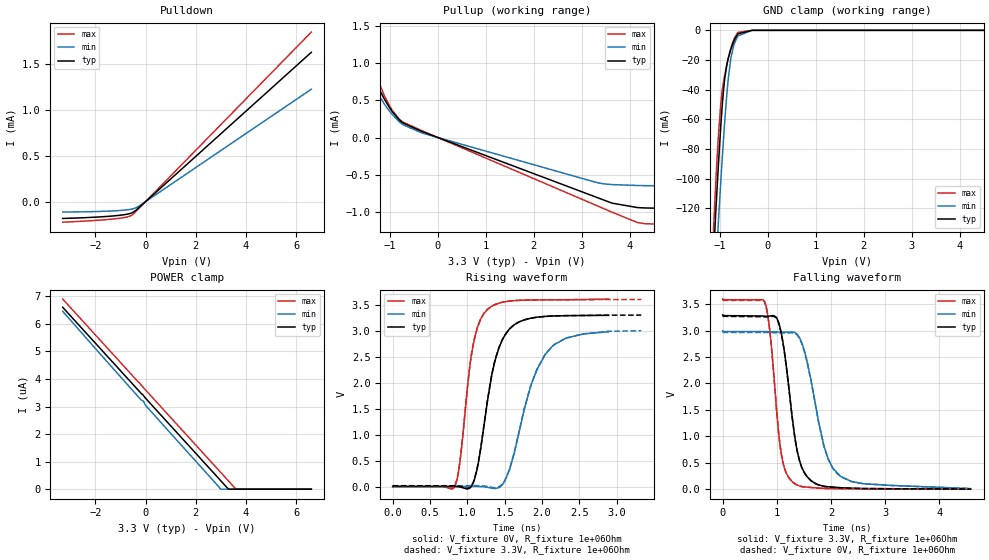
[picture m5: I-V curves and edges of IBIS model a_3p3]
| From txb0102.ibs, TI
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|   a_3p3 Model
[Model]   a_3p3
Model_type   I/O
Polarity   Non-Inverting
Enable   Active-High
Vinl = 1.155
Vinh = 2.145
Vmeas = 1.65
Vref = 0
Cref = 2pF
Rref = 1e6
|   typ   min   max
|   (nom PVT)   (fast PVT)   (slow PVT)
C_comp   3.766e-12   3.694e-12   3.795e-12
[Model spec]
|subparameter
Vinl   1.155   1.05   1.26
Vinh   2.145   1.95   2.34
| Where nom  PVT is Nominal Process, 3.3V, 27C
|   Fast PVT is Strong Process,  3.6V, -40C
|   Slow PVT is Weak Process,   3V, 125C
[Voltage Range]   3.3   3   3.6
|Junction Temperature
[Temperature Range]   27   125   -40
[Pullup Reference]   3.3   3   3.6
[Pulldown Reference]   0   0   0
[Power Clamp Reference]   3.3   3   3.6
[GND Clamp Reference]   0   0   0
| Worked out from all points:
|   slope of the pulldown table from 0 to 0.495 V, typ, clamps not added: 4.05 kohm
|   slope of the pullup table from 0 to 0.495 V, typ, clamps not added: 4.1 kohm
|   falling waveform, V_fixture 3.3V, R_fixture 1e+06Ohm: 20-80 % time 256ps typ, 373ps min, 193ps max; typ from 3.3 V to -0.003 V
|   rising waveform, V_fixture 0V, R_fixture 1e+06Ohm: 20-80 % time 245ps typ, 363ps min, 183ps max; typ from 0 V to 3.3 V
|   rising waveform, V_fixture 3.3V, R_fixture 1e+06Ohm: 20-80 % time 246ps typ, 368ps min, 181ps max; typ from 0.013 V to 3.3 V
|   falling waveform, V_fixture 0V, R_fixture 1e+06Ohm: 20-80 % time 254ps typ, 371ps min, 192ps max; typ from 3.27 V to -0.003 V
[Pulldown]
|   Voltage   I(typ)   I(min)   I(max)
-3.3V     -183.7uA   -113.8uA   -224.3uA
-1.262V   -155.6uA   -100.8uA   -188.7uA
-729.3mV  -136.7uA   -89.39uA   -167.2uA
-508.2mV  -117.6uA   -78.82uA   -139.8uA
-204.6mV  -50.47uA   -37.88uA   -57.3uA
6.6V      1.627mA    1.225mA    1.848mA
[GND Clamp]
|   Voltage   I(typ)   I(min)   I(max)
-3.3V     -1.793A    -1.701A    -1.88A
-1.216V   -205.9mA   -237.9mA   -190.6mA
-1.093V   -127.4mA   -164.5mA   -107.6mA
-1.068V   -112.3mA   -150mA     -92.06mA
-1.028V   -89.41mA   -127.7mA   -69.86mA
-976.8mV  -62.43mA   -99.84mA   -47.8mA
-891.6mV  -30.76mA   -58.31mA   -28.87mA
-831mV    -19.69mA   -34.58mA   -19.53mA
-772.8mV  -12.86mA   -18.99mA   -12.11mA
-618mV    -2.313mA   -3.709mA   -1.329mA
-315mV    -2.259uA   -24.11uA   -369.2nA
6.6V      0A         0A         0A
[Pullup]
|   Voltage   I(typ)   I(min)   I(max)
-3.3V     6.744mA    4.882mA    9.601mA
-1.806V   1.679mA    1.67mA     1.956mA
-1.704V   1.443mA    1.387mA    1.703mA
-1.536V   1.123mA    1.009mA    1.321mA
-1.495V   1.053mA    934.4uA    1.235mA
-1.373V   860.4uA    744.5uA    992.1uA
-1.115V   518.3uA    450.8uA    565.8uA
-801.6mV  236.6uA    211.4uA    245.2uA
-330mV    80.49uA    60.75uA    91.57uA
3.324V    -811uA     -608.8uA   -922.5uA
4.161V    -945.6uA   -647.7uA   -1.147mA
6.6V      -979.1uA   -657.1uA   -1.212mA
[POWER Clamp]
|   Voltage   I(typ)   I(min)   I(max)
-3.3V     6.601uA    6.456uA    6.901uA
-283.2mV  3.584uA    3.346uA    3.885uA
-165mV    3.466uA    3.233uA    3.769uA
-93mV     3.41uA     3.202uA    3.693uA
-23.1mV   3.324uA    3.076uA    3.623uA
46.2mV    3.254uA    2.995uA    3.554uA
2.988V    312nA      0A         612nA
3.303V    0A         0A         296.7nA
3.598V    0A         0A         0A
6.6V      0A         0A         0A
[Ramp]
R_load = 1e+06
|   typ   min   max
dV/dt_r   1.96825/2.41762e-10   1.7882/3.57035e-10   2.14772/1.77444e-10
dV/dt_f   1.96601/2.52716e-10   1.78466/3.69251e-10   2.14592/1.89729e-10
[Falling Waveform]
V_fixture = 3.3V
V_fixture_min = 3V
V_fixture_max = 3.6V
R_fixture = 1e+06Ohm
|   Time   V(typ)   V(min)   V(max)
0s        3.3V       3V         3.6V
774ps     3.276V     2.983V     3.553V
866ps     3.277V     2.982V     3.035V
1.08ns    2.962V     2.972V     679.6mV
1.328ns   1.009V     2.968V     100.6mV
1.42ns    532.2mV    2.862V     55.52mV
1.558ns   233.2mV    2.422V     33.89mV
1.872ns   50.43mV    808.2mV    10.7mV
2.174ns   23.79mV    240.3mV    4.942mV
4.542ns   -2.624mV   8.57mV     -4.623mV
[Rising Waveform]
V_fixture = 0V
V_fixture_min = 0V
V_fixture_max = 0V
R_fixture = 1e+06Ohm
|   Time   V(typ)   V(min)   V(max)
0s        253.9nV    70.12uV    51.49nV
832ps     1.653mV    -110.2uV   -1.142mV
902ps     -9.455mV   -38.98uV   486.9mV
1.08ns    73.73mV    1.276mV    2.741V
1.268ns   1.637V     -15.06mV   3.409V
1.364ns   2.386V     -39.18mV   3.498V
1.502ns   2.912V     105.1mV    3.557V
1.844ns   3.239V     1.909V     3.591V
2.044ns   3.275V     2.543V     3.594V
2.89ns    3.296V     2.978V     3.609V
[Rising Waveform]
V_fixture = 3.3V
V_fixture_min = 3V
V_fixture_max = 3.6V
R_fixture = 1e+06Ohm
|   Time   V(typ)   V(min)   V(max)
0s        13.27mV    16.03mV    12.76mV
832ps     14.92mV    15.85mV    11.77mV
902ps     3.818mV    15.92mV    500mV
1.026ns   -23.78mV   16.75mV    2.239V
1.096ns   153.2mV    17.38mV    2.855V
1.32ns    2.104V     -13.73mV   3.466V
1.562ns   3.033V     327.1mV    3.57V
1.864ns   3.245V     2.006V     3.592V
2.13ns    3.282V     2.691V     3.594V
3.33ns    3.3V       3V         3.6V
[Falling Waveform]
V_fixture = 0V
V_fixture_min = 0V
V_fixture_max = 0V
R_fixture = 1e+06Ohm
|   Time   V(typ)   V(min)   V(max)
0s        3.273V     2.967V     3.574V
774ps     3.263V     2.967V     3.54V
866ps     3.264V     2.966V     3.022V
1.08ns    2.95V      2.956V     674mV
1.328ns   1.002V     2.952V     99.54mV
1.418ns   534.9mV    2.85V      55.6mV
1.556ns   231.7mV    2.415V     33.85mV
1.87ns    47.98mV    806.5mV    10.65mV
2.174ns   22.63mV    236.8mV    4.857mV
4.591ns   -2.726mV   8.29mV     -4.644mV
